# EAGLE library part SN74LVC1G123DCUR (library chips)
Monostable Multivibrator
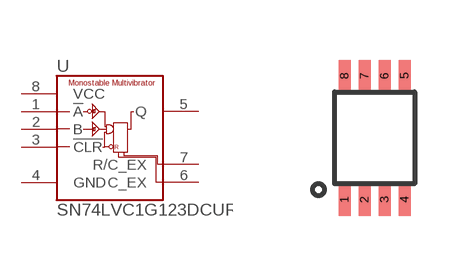
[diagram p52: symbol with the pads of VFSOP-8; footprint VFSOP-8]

Designator prefix U

## SN74LVC1G123DCUR (DIGIKEY: 296-18578-1-ND)  [VFSOP-8]
1  !A
2  B
3  !CLR
4  GND
5  Q
6  C_EX
7  R/C_EX
8  VCC

## Footprint VFSOP-8 (pad centres in mm)
smd 0.3 x 0.8: 1 -0.75,-1.55; 2 -0.25,-1.55; 3 0.25,-1.55; 4 0.75,-1.55; 5 0.75,1.55; 6 0.25,1.55; 7 -0.25,1.55; 8 -0.75,1.55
